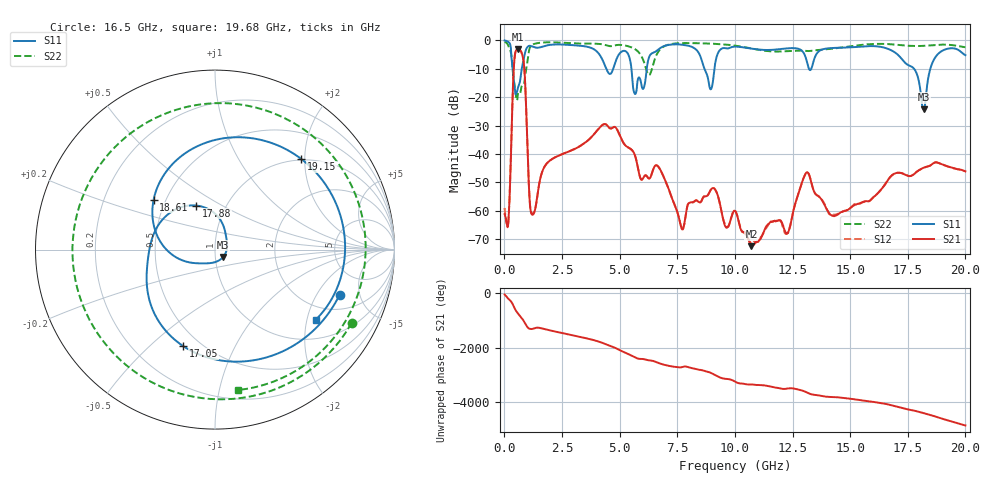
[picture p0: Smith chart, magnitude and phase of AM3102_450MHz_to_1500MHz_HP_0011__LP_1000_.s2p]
!Agilent Technologies,E8364B,MY43040894,A.07.50.67
!Agilent E8364B: A.07.50.67
!Date: Thursday, January 11, 2018 05:32:12
!Correction: S11(Full 2 Port(1,2))
!S21(Full 2 Port(1,2))
!S12(Full 2 Port(1,2))
!S22(Full 2 Port(1,2))
!S2P File: Measurements: S11, S21, S12, S22:
# Hz S  dB  R 50
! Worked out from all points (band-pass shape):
!   1601 points, 10 MHz to 20 GHz, reference 50 ohm
!   highest |S21| = -3.13 dB at 584.7 MHz (marker M1); lowest = -72.4 dB at 10.72 GHz (marker M2)
!   |S21| within 3 dB of the highest: 442.6 MHz to 806 MHz (363.3 MHz wide, 58.2 % of centre)
!   lowest |S11| = -24.3 dB at 18.19 GHz (marker M3), VSWR 1.13, Z = 54.5 - j4.53 ohm
!   |S11| at or under -10 dB: 5.512 GHz to 6.176 GHz (663.9 MHz wide, 11.4 % of centre); 8.679 GHz to 9.111 GHz (431.5 MHz wide, 4.85 % of centre); 17.77 GHz to 18.48 GHz (707.2 MHz wide, 3.9 % of centre)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
!   |S22| runs from -21.2 to -0.5 dB; largest |S21 - S12| = 0.0025
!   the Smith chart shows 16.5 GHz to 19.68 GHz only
!   S11 on the Smith chart (normalised r, x): 16.5 GHz: 2.90, -3.21; 17.05 GHz: 0.41, -0.64; 17.88 GHz: 0.73, +0.38; 18.61 GHz: 0.43, +0.30; 19.15 GHz: 0.98, +1.93; 19.68 GHz: 1.55, -2.27
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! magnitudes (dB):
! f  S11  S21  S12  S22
! 10 MHz  -0.1  -61.1  -59.0  -0.5
! 172.4 MHz  -0.6  -64.2  -63.9  -1.9
! 422.3 MHz  -15.1  -8.0  -8.0  -14.6
! 584.7 MHz  -16.9  -3.1  -3.1  -19.0
! 834.6 MHz  -6.7  -7.5  -7.5  -15.4
! 1.209 GHz  -2.2  -61.4  -61.0  -1.6
! 3.346 GHz  -2.0  -36.9  -36.9  -1.1
! 5.657 GHz  -18.8  -40.3  -40.3  -3.1
! 6.682 GHz  -3.2  -44.5  -44.5  -4.0
! 7.706 GHz  -1.6  -66.5  -66.5  -1.0
! 10.01 GHz  -2.2  -60.1  -60.0  -1.9
! 10.72 GHz  -2.9  -72.4  -70.9  -2.9
! 13.34 GHz  -9.5  -50.9  -50.8  -3.7
! 16.5 GHz  -2.6  -50.9  -50.7  -1.3
! 16.68 GHz  -3.1  -48.7  -48.7  -1.3
! 17.05 GHz  -4.9  -46.6  -46.6  -1.6
! 17.88 GHz  -11.5  -46.4  -46.3  -2.0
! 18.19 GHz  -24.3  -44.8  -44.8  -1.9
! 18.61 GHz  -7.1  -43.2  -43.3  -1.7
! 19.15 GHz  -3.1  -44.2  -44.2  -1.5
! 19.68 GHz  -3.3  -45.4  -45.4  -2.0
! 20 GHz  -5.2  -46.1  -46.0  -2.4
